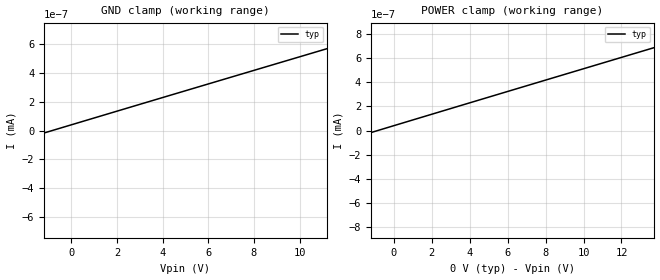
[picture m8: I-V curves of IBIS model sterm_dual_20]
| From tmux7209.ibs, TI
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| sterm_dual_20
[Model]   sterm_dual_20
Model_type   Terminator
|   typ   min   max
C_comp   1.008417e-11   NA   NA
[Voltage Range]   0   -20   20
[Temperature Range]   27   NA   NA
[Power Clamp Reference]   0   NA   NA
[GND Clamp Reference]   0   NA   NA
[GND Clamp]
|   Voltage   I(typ)   I(min)   I(max)
-25V      -1.609A    NA         NA
-15.91V   -724.8pA   NA         NA
-909.1mV  -3.331pA   NA         NA
14.09V    703.6pA    NA         NA
14.55V    724.9pA    NA         NA
20V       982.4pA    NA         NA
[POWER Clamp]
|   Voltage   I(typ)   I(min)   I(max)
-20V      -926.2pA   NA         NA
-18.64V   -858.2pA   NA         NA
-3.182V   -111.4pA   NA         NA
17.27V    853pA      NA         NA
17.73V    874.3pA    NA         NA
25V       3.307A     NA         NA
